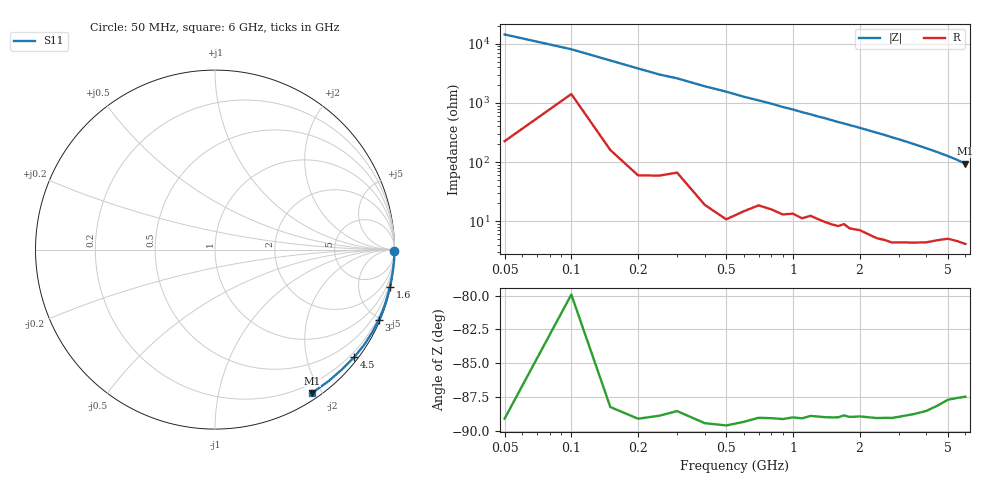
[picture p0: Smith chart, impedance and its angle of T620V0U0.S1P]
! SIEMENS Discrete & RF Semiconductors
! BAT62
! Si Schottky Diode in SOT143
! VR = 20 V
! S-Parameters:  February  1997
# GHz  S  MA  R  50
!  f  S11
! GHz  MAG  ANG
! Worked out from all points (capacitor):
!   34 points, 50 MHz to 6 GHz, reference 50 ohm
!   read as one part to ground: C = 204 fF near 50 MHz
!   lowest |Z| = 94.2 ohm at 6 GHz (marker M1)
!   S11 on the Smith chart (normalised r, x): 50 MHz: open; 1.6 GHz: 0.17, -9.51; 3 GHz: 0.09, -4.87; 4.5 GHz: 0.10, -2.93; 6 GHz: 0.08, -1.88
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0.05  0.9999 -0.4
0.1  0.9978 -0.7
0.15  0.9994 -1.1
0.2  0.9996 -1.5
0.3  0.999 -2.2
0.5  0.9996 -3.7
0.6  0.9991 -4.5
0.8  0.9983 -5.9
0.9  0.9982 -6.7
1  0.9978 -7.4
1.1  0.9977 -8.2
1.2  0.997 -8.9
1.3  0.9969 -9.7
1.4  0.9968 -10.4
1.6  0.9964 -12.0
1.7  0.9956 -12.7
1.8  0.9958 -13.5
1.9  0.9955 -14.2
2.4  0.9949 -18.2
2.6  0.9943 -19.8
2.8  0.9939 -21.6
3  0.9929 -23.2
3.5  0.99 -27.7
4  0.9862 -32.5
4.5  0.9802 -37.6
5  0.9729 -43.1
5.5  0.9684 -49.1
6  0.9642 -55.9
